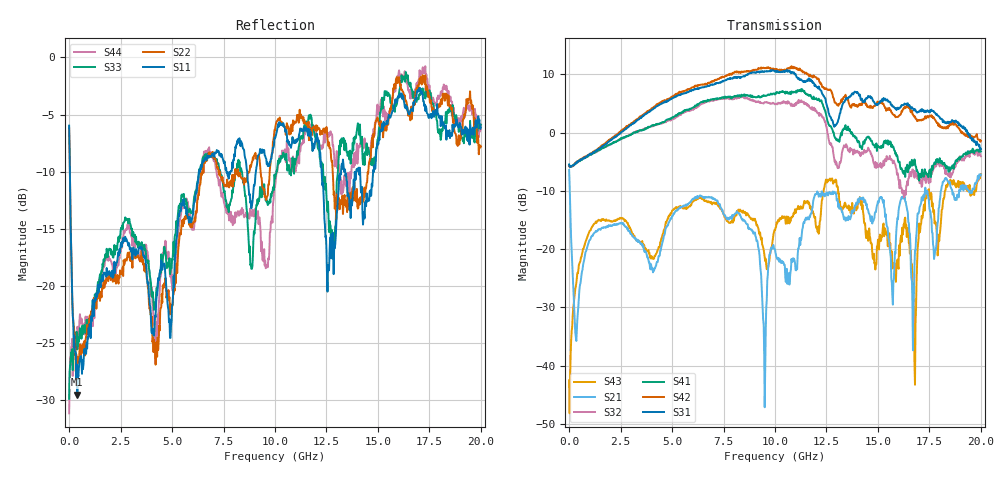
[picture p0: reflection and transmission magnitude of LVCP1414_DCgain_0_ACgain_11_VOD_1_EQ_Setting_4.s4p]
!Agilent Technologies,N5230A,MY46400459,A.07.50.48
!Agilent N5230A: A.07.50.48
!Date: Tuesday, April 17, 2012 18:30:58
!Correction: S11(Full 4 Port(1,2,3,4))
!S12(Full 4 Port(1,2,3,4))
!S13(Full 4 Port(1,2,3,4))
!S14(Full 4 Port(1,2,3,4))
!S21(Full 4 Port(1,2,3,4))
!S22(Full 4 Port(1,2,3,4))
!S23(Full 4 Port(1,2,3,4))
!S24(Full 4 Port(1,2,3,4))
!S31(Full 4 Port(1,2,3,4))
!S32(Full 4 Port(1,2,3,4))
!S33(Full 4 Port(1,2,3,4))
!S34(Full 4 Port(1,2,3,4))
!S41(Full 4 Port(1,2,3,4))
!S42(Full 4 Port(1,2,3,4))
!S43(Full 4 Port(1,2,3,4))
!S44(Full 4 Port(1,2,3,4))
!S4P File: Measurements: <S11,S12,S13,S14>,
!<S21,S22,S23,S24>,
!<S31,S32,S33,S34>,
!<S41,S42,S43,S44>:
# Hz S  dB  R 50
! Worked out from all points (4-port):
!   801 points, 300 kHz to 20 GHz, reference 50 ohm
!   strongest paths, dB at 300 kHz, 5 GHz, 10 GHz, 15 GHz, 20 GHz:
!     S31: -5.5, 5.9, 10.5, 4.8, -2.8
!     S42: -5.7, 6.2, 10.8, 5.2, -1.4
!     S41: -5.5, 2.6, 6.5, -2.4, -3.2
!     S32: -5.6, 2.3, 4.9, -5.9, -4.1
!     S21: -6.4, -14.3, -20.0, -11.8, -7.2
!     S43: -42.5, -13.4, -16.8, -18.4, -7.1
!   lowest |S11| = -29.5 dB at 400.3 MHz (marker M1), VSWR 1.07, Z = 53.1 + j1.54 ohm
!   |S11| at or under -10 dB: 37.67 MHz to 6.317 GHz (6.279 GHz wide, 198 % of centre); 12.27 GHz to 13.21 GHz (942.3 MHz wide, 7.4 % of centre); 14.13 GHz to 14.77 GHz (635.9 MHz wide, 4.4 % of centre)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
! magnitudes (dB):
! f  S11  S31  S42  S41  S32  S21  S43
! 300 kHz  -6.0  -5.5  -5.7  -5.5  -5.6  -6.4  -42.5
! 400.3 MHz  -29.5  -5.0  -4.9  -5.1  -5.0  -32.0  -24.1
! 10.05 GHz  -6.8  10.5  10.8  6.7  4.9  -21.0  -16.2
! 12.7 GHz  -15.7  2.7  7.3  1.1  -2.1  -10.5  -8.2
! 16.78 GHz  -3.9  4.0  2.7  -4.6  -7.7  -22.9  -39.6
! 17.4 GHz  -4.9  3.8  2.9  -7.3  -7.7  -10.0  -10.2
! 20 GHz  -6.1  -2.8  -1.4  -3.2  -4.1  -7.2  -7.1
